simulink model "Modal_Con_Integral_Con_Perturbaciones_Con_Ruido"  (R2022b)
settings: Solver=ode4  StartTime=0.0  StopTime=0.2  FixedStep=1e-6  RelTol=1e-3
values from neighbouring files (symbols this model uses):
  A = [-R_1/L_1,  omega_1    [Modal_Integral.m]    (also in PI_Lazo_V_DC.m = -10000; LQR_Sin_Integral.m; LQR_Con_Integral.m)
  B = [-V_DC0/(2*L_1*m_t1),  0    [Modal_Integral.m]    (also in PI_Lazo_V_DC.m = 10000; LQR_Sin_Integral.m; LQR_Con_Integral.m)
  C = eye(2)    [Modal_Integral.m]    (also in PI_Lazo_V_DC.m = 1; LQR_Sin_Integral.m; LQR_Con_Integral.m)
  D = zeros(2)    [Modal_Integral.m]    (also in PI_Lazo_V_DC.m = 0; LQR_Sin_Integral.m; LQR_Con_Integral.m)
  Delta_v_d_1 = 8    [Modal_Integral.m]    (also in IP_Lazo_Q_12.m = P_Delta_v_d_1*v_d_12; LQR_Con_Integral.m)
  Delta_v_q_1 = 1    [Modal_Integral.m]    (also in LQR_Con_Integral.m)
  E = [1/L_1,  0    [Modal_Integral.m]    (also in LQR_Sin_Integral.m; LQR_Con_Integral.m)
  I_Delta_v_1 = 0.1    [Modal_Integral.m]    (also in LQR_Con_Integral.m)
  I_p_1 = 0.15    [Modal_Integral.m]    (also in LQR_Con_Integral.m)
  Kc = Kca_place(:, 1:2)    [Modal_Integral.m]    (also in LQR_Con_Integral.m = Kca(:, 1:2))
  Ki = -Kca_place(:, 3:4)    [Modal_Integral.m]    (also in LQR_Con_Integral.m = -Kca(:, 3:4))
  p_11 = 5    [Modal_Integral.m]    (also in LQR_Con_Integral.m)
  p_12 = -2    [Modal_Integral.m]    (also in LQR_Con_Integral.m)
  tau = te    (= 0.001)    [Modal_Integral.m]    (also in IP_Lazo_P_2.m = 0.002; IP_Lazo_Q_12.m = 0.002; LQR_Sin_Integral.m = 0.002; LQR_Con_Integral.m)
  v_d_1 = 100*sqrt(2)    [Modal_Integral.m]    (also in PI_Lazo_V_DC.m; LQR_Sin_Integral.m; LQR_Con_Integral.m; Sistema_no_lineal_Modal.m)
  v_q_1 = 0    [Modal_Integral.m]    (also in LQR_Sin_Integral.m; LQR_Con_Integral.m)
  V_R_i = D_R_i^2    (= 2.5e-05)    [Modal_Integral.m]    (also in LQR_Con_Integral.m; Sistema_no_lineal_Modal.m; Sistema_no_lineal_LQR.m; Sistema_control_no_lineal_LQR.m)
  W = [1,  0    [Modal_Integral.m]    (also in LQR_Con_Integral.m)

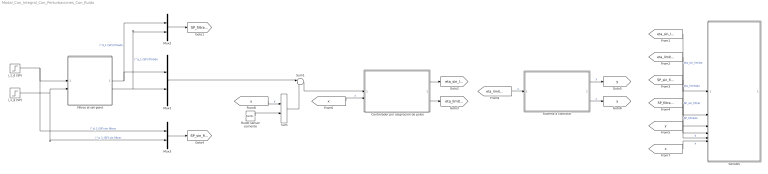
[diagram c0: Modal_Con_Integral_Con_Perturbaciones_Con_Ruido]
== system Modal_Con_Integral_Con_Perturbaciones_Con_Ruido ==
  Controlador por asignación de polos : Subsystem
  Filtros al set-point : Subsystem
  Mux1 : Mux  Inputs=2
  Mux2 : Mux  Inputs=2
  Mux3 : Mux  Inputs=2
  Ruido sensor corriente : RandomNumber  Variance=V_R_i  SampleTime=0.001
  Señales : Subsystem
  Sistema a controlar : Subsystem
  Sum : Sum
  Sum1 : Sum  Inputs=|+-
  i_1_d (SP) : Step  Time=0.05  Before=18  After=-2  SampleTime=0
  i_1_q (SP) : Step  Time=0.05  Before=-15  After=-5  SampleTime=0
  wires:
  Mux2/1 -> [SP_filtrado]
  Sistema a controlar/1(y) -> [y]  "y"
  Sistema a controlar/2(x) -> [x]  "x"
  i_1_d (SP)/1 -> Mux3/1, Filtros al set-point/1(i_1_d sin filtrar)  "i^d_1 (SP) sin filtrar"
  i_1_q (SP)/1 -> Mux3/2, Filtros al set-point/2(i_1_q sin filtrar)  "i^q_1 (SP) sin filtrar"
  Mux3/1 -> [SP_sin_filtrar]
  [eta_sin_limitar] -> Señales/1(eta_sin_limitar)  "eta_sin_limitar"
  [eta_limitado] -> Señales/2(eta_limitado)  "eta_limitado"
  [SP_sin_filtrar] -> Señales/3(SP_sin_filtrar)  "SP_sin_filtrar"
  [SP_filtrado] -> Señales/4(SP_filtrado)  "SP_filtrado"
  [y] -> Señales/5(y)  "y"
  [x] -> Señales/6(x)  "x"
  Filtros al set-point/1(i_1_d filtrado) -> Mux2/1, Mux1/1  "i^d_1 (SP) filtrado"
  Filtros al set-point/2(i_1_q filtrado) -> Mux1/2, Mux2/2  "i^q_1 (SP) filtrado"
  [y] -> Sum/1  "y"
  Controlador por asignación de polos/2(eta limitado) -> [eta_limitado]
  Sum1/1 -> Controlador por asignación de polos/1(e)
  Controlador por asignación de polos/1(eta sin limitar) -> [eta_sin_limitar]
  [x] -> Controlador por asignación de polos/2(x)  "x"
  [eta_limitado] -> Sistema a controlar/1(u)  "u"
  Mux1/1 -> Sum1/1
  Sum/1 -> Sum1/2
  Ruido sensor corriente/1 -> Sum/2

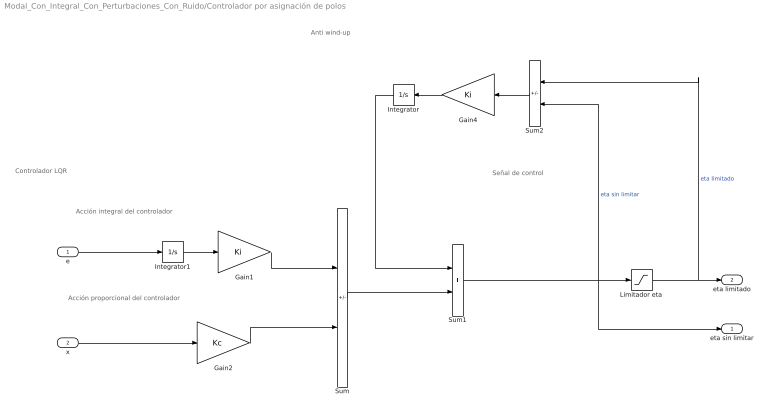
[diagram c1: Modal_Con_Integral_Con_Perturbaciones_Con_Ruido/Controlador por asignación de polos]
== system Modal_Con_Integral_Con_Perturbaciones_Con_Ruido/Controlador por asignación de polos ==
  note: Señal de control
  note: Anti wind-up
  note: Controlador LQR
  note: Acción proporcional del controlador
  note: Acción integral del controlador
  e : Inport
  x : Inport  Port=2
  Gain1 : Gain  Gain=Ki  Multiplication=Matrix(K*u) (u vector)
  Gain2 : Gain  Gain=Kc  Multiplication=Matrix(K*u) (u vector)
  Gain4 : Gain  Gain=Ki  Multiplication=Matrix(K*u) (u vector)
  Integrator : Integrator
  Integrator1 : Integrator
  Limitador eta : Saturate  UpperLimit=5  LowerLimit=-5
  Sum : Sum  Inputs=+-
  Sum1 : Sum
  Sum2 : Sum  Inputs=+-
  eta sin limitar : Outport
  eta limitado : Outport  Port=2
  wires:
  Gain1/1 -> Sum/1
  x/1 -> Gain2/1
  Gain2/1 -> Sum/2
  Limitador eta/1 -> eta limitado/1, Sum2/1  "eta limitado"
  e/1 -> Integrator1/1
  Integrator/1 -> Sum1/1
  Sum2/1 -> Gain4/1
  Sum1/1 -> eta sin limitar/1, Sum2/2, Limitador eta/1  "eta sin limitar"
  Gain4/1 -> Integrator/1
  Integrator1/1 -> Gain1/1
  Sum/1 -> Sum1/2

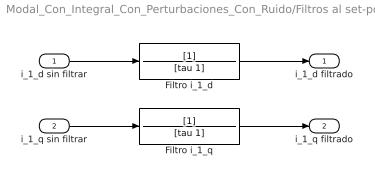
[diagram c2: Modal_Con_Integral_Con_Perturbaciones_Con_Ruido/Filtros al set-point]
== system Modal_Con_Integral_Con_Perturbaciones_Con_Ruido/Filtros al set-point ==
  i_1_d sin filtrar : Inport
  i_1_q sin filtrar : Inport  Port=2
  Filtro i_1_d : TransferFcn  Denominator=[tau 1]
  Filtro i_1_q : TransferFcn  Denominator=[tau 1]
  i_1_d filtrado : Outport
  i_1_q filtrado : Outport  Port=2
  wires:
  i_1_q sin filtrar/1 -> Filtro i_1_q/1
  i_1_d sin filtrar/1 -> Filtro i_1_d/1
  Filtro i_1_d/1 -> i_1_d filtrado/1
  Filtro i_1_q/1 -> i_1_q filtrado/1

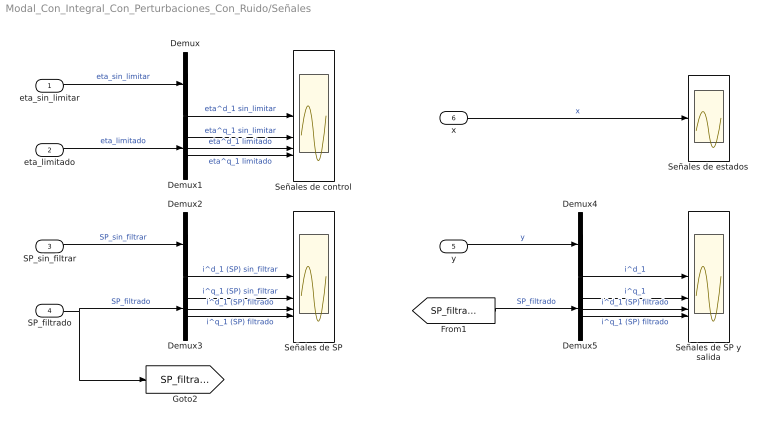
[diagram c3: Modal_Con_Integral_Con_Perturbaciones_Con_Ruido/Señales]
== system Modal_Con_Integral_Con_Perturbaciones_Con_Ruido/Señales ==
  eta_sin_limitar : Inport
  eta_limitado : Inport  Port=2
  SP_sin_filtrar : Inport  Port=3
  SP_filtrado : Inport  Port=4
  y : Inport  Port=5
  x : Inport  Port=6
  Demux{,1..5} (6 alike) : Demux  Outputs=2
  Señales de SP : Scope  NumInputPorts=4
  Señales de SP y salida : Scope  NumInputPorts=4
  Señales de control : Scope  NumInputPorts=4
  Señales de estados : Scope
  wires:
  y/1 -> Demux4/1  "y"
  eta_sin_limitar/1 -> Demux/1  "eta_sin_limitar"
  SP_filtrado/1 -> [SP_filtrado], Demux3/1  "SP_filtrado"
  x/1 -> Señales de estados/1  "x"
  SP_sin_filtrar/1 -> Demux2/1  "SP_sin_filtrar"
  eta_limitado/1 -> Demux1/1  "eta_limitado"
  [SP_filtrado] -> Demux5/1  "SP_filtrado"
  Demux1/2 -> Señales de control/4  "eta^q_1 limitado"
  Demux/1 -> Señales de control/1  "eta^d_1 sin_limitar"
  Demux/2 -> Señales de control/2  "eta^q_1 sin_limitar"
  Demux1/1 -> Señales de control/3  "eta^d_1 limitado"
  Demux3/1 -> Señales de SP/3  "i^d_1 (SP) filtrado"
  Demux3/2 -> Señales de SP/4  "i^q_1 (SP) filtrado"
  Demux2/2 -> Señales de SP/2  "i^q_1 (SP) sin_filtrar"
  Demux2/1 -> Señales de SP/1  "i^d_1 (SP) sin_filtrar"
  Demux4/1 -> Señales de SP y salida/1  "i^d_1"
  Demux4/2 -> Señales de SP y salida/2  "i^q_1"
  Demux5/2 -> Señales de SP y salida/4  "i^q_1 (SP) filtrado"
  Demux5/1 -> Señales de SP y salida/3  "i^d_1 (SP) filtrado"

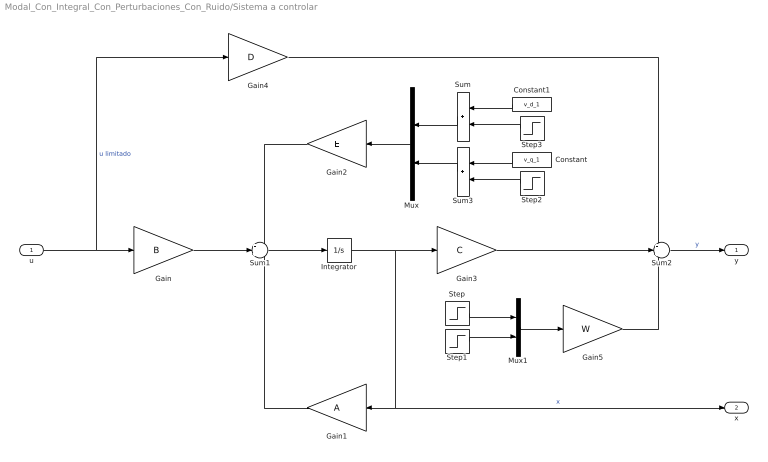
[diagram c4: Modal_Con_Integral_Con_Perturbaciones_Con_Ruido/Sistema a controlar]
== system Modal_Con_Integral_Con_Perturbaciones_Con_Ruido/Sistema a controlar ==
  u : Inport
  Constant : Constant  Value=v_q_1
  Constant1 : Constant  Value=v_d_1
  Gain : Gain  Gain=B  Multiplication=Matrix(K*u) (u vector)
  Gain1 : Gain  Gain=A  Multiplication=Matrix(K*u) (u vector)
  Gain2 : Gain  Gain=E  Multiplication=Matrix(K*u) (u vector)
  Gain3 : Gain  Gain=C  Multiplication=Matrix(K*u) (u vector)
  Gain4 : Gain  Gain=D  Multiplication=Matrix(K*u) (u vector)
  Gain5 : Gain  Gain=W  Multiplication=Matrix(K*u) (u vector)
  Integrator : Integrator
  Mux : Mux  Inputs=2
  Mux1 : Mux  Inputs=2
  Step : Step  Time=I_p_1  After=p_11  SampleTime=0
  Step1 : Step  Time=I_p_1  After=p_12  SampleTime=0
  Step2 : Step  Time=I_Delta_v_1  After=Delta_v_q_1  SampleTime=0
  Step3 : Step  Time=I_Delta_v_1  After=Delta_v_d_1  SampleTime=0
  Sum : Sum
  Sum1 : Sum  Inputs=+++
  Sum2 : Sum  Inputs=+++
  Sum3 : Sum
  y : Outport
  x : Outport  Port=2
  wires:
  Gain/1 -> Sum1/2
  Gain1/1 -> Sum1/3
  Integrator/1 -> x/1, Gain1/1, Gain3/1  "x"
  Sum2/1 -> y/1  "y"
  Sum1/1 -> Integrator/1
  Gain3/1 -> Sum2/2
  Gain4/1 -> Sum2/1
  u/1 -> Gain4/1, Gain/1  "u limitado"
  Mux/1 -> Gain2/1
  Constant1/1 -> Sum/1
  Constant/1 -> Sum3/1
  Gain2/1 -> Sum1/1
  Mux1/1 -> Gain5/1
  Step/1 -> Mux1/1
  Step1/1 -> Mux1/2
  Gain5/1 -> Sum2/3
  Sum/1 -> Mux/1
  Sum3/1 -> Mux/2
  Step2/1 -> Sum3/2
  Step3/1 -> Sum/2
